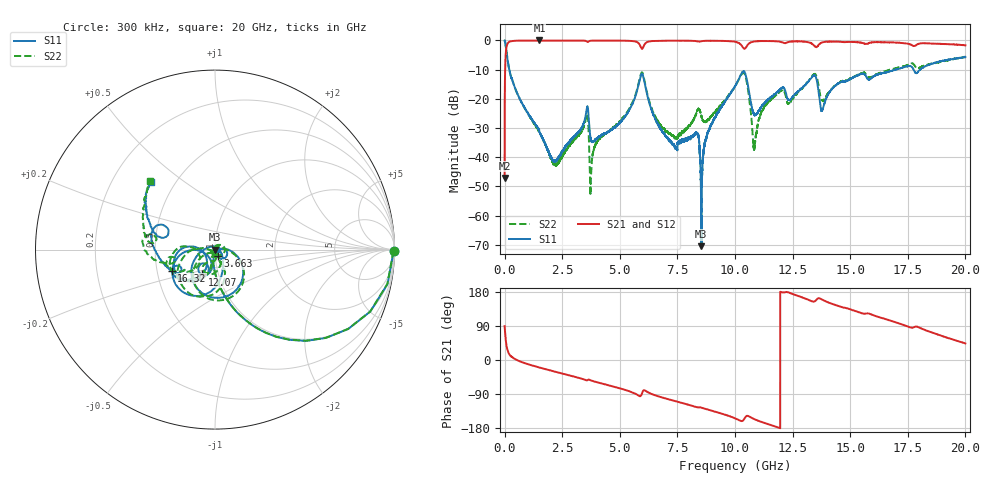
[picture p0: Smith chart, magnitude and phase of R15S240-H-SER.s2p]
!{R15S240}
!Johanson Technology Inc.
!www.johansontechnology.com
!Test Board Conditions:
!Substrate Type  RO4350B
!Substrate Thickness  20 mil
!Substrate Dk  3.66
!TL Type: GCPW
!TL Trace Width  34 mil
!TL Gap  10 mil
!Electrode orientation  Horizontal
!DUT TOPOLOGY	SERIES
!Mounting Pad LxW  26x52 mil
! Created Sat Feb  6 14:23:17 2021
# hz S ma R 50
! 2 Port Network Data from SP1.SP block
! freq  magS11  angS11  magS21  angS21  magS12  angS12  magS22  angS22
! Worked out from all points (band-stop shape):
!   20001 points, 300 kHz to 20 GHz, reference 50 ohm
!   highest |S21| = -0.01 dB at 1.512 GHz (marker M1); lowest = -47.1 dB at 300 kHz (marker M2)
!   |S21| within 3 dB of the highest: 67.88 MHz to end of sweep
!   lowest |S11| = -70.5 dB at 8.537 GHz (marker M3), VSWR 1.00, Z = 50 - j0.00628 ohm
!   |S11| at or under -10 dB: 202.5 MHz to 16.96 GHz (16.76 GHz wide, 195 % of centre); 16.96539 GHz to 16.97053 GHz (5.139 MHz wide, 0.0303 % of centre); 17.75 GHz to 18.04 GHz (288 MHz wide, 1.61 % of centre)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
!   |S22| runs from -52.6 to 0.0 dB; largest |S21 - S12| = 0.017
!   S11 on the Smith chart (normalised r, x): 300 kHz: open; 3.663 GHz: 1.03, -0.08; 12.07 GHz: 0.83, -0.24; 16.32 GHz: 0.60, -0.15; 20 GHz: 0.37, +0.38
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300000  0.9956 -0.4  0.004434 89.3  0.004364 89.8  0.9947 -0.4
1.563e8  0.3951 -68.9  0.9151 21.1  0.9166 20.9  0.3974 -68.6
1.5123e9  0.02696 -101.5  0.9993 -19.9  0.9983 -19.8  0.02678 -116.3
2.2033e9  0.008695 -40.8  0.9983 -31.1  0.997 -31.0  0.007645 168.6
3.3343e9  0.03113 8.3  0.9939 -49.1  0.9941 -49.2  0.02732 64.1
3.5533e9  0.06296 -5.3  0.9682 -53.6  0.9686 -53.6  0.05085 21.6
3.6633e9  0.03969 -69.3  0.9699 -51.9  0.9696 -51.9  0.01871 -83.8
4.8613e9  0.03504 4.8  0.9923 -72.5  0.9923 -72.5  0.03644 21.8
5.9503e9  0.2696 -78.6  0.7201 -90.2  0.7214 -90.1  0.2838 -76.9
6.6673e9  0.03606 158.3  0.9867 -95.7  0.9856 -95.7  0.04103 -150.5
8.3373e9  0.02584 -29.3  0.9701 -124.5  0.9697 -124.4  0.05857 -88.2
8.5373e9  0.0002995 -167.9  0.9699 -125.7  0.9692 -125.6  0.0511 -115.7
8.8823e9  0.02942 -15.3  0.9857 -131.9  0.9862 -131.9  0.04517 -82.9
1.00003e10  0.1646 -79.3  0.951 -153.7  0.9508 -153.7  0.1643 -69.9
1.04343e10  0.2788 -148.1  0.7246 -152.0  0.7265 -152.1  0.2586 -141.7
1.08523e10  0.05296 -142.8  0.9607 -156.5  0.9615 -156.4  0.01522 -104.6
1.20723e10  0.1567 -117.8  0.9201 178.2  0.9219 178.2  0.1435 -107.9
1.33343e10  0.2344 -131.7  0.8828 155.0  0.8853 154.9  0.2393 -134.9
1.37893e10  0.06412 -141.9  0.9268 159.1  0.9285 159.0  0.0932 -162.6
1.63203e10  0.269 -154.3  0.9351 111.7  0.9271 111.7  0.2822 -164.2
1.66673e10  0.2917 -163.8  0.9298 105.4  0.9175 105.2  0.3105 -166.8
2e10  0.517 133.6  0.8253 43.7  0.8167 43.4  0.5269 133.1
